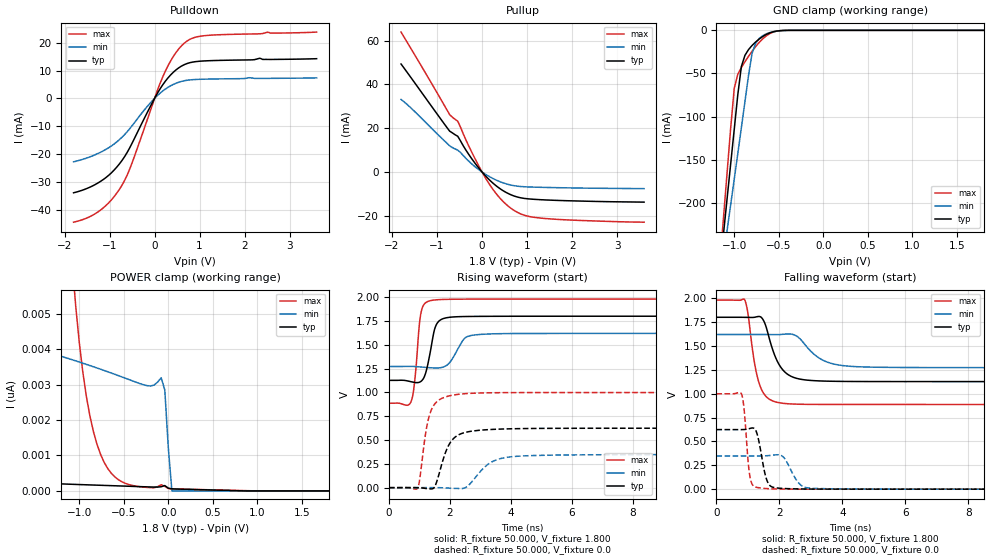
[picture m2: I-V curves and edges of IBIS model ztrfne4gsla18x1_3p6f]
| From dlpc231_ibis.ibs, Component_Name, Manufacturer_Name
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| Model ztrfne4gsla18x1_3p6f
[Model] ztrfne4gsla18x1_3p6f
Model_type I/O
Polarity   Non-Inverting
Enable   Active-High
Vinl =  0.540V
Vinh =  1.260V
Vref = 0.000V
Rref = 0.50k
Cref = 50.00pF
Vmeas = 0.90V
C_comp   2.222pF   2.219pF   2.262pF
C_comp_pullup   0.543pF   0.497pF   0.685pF
C_comp_pulldown   0.543pF   0.497pF   0.685pF
[Temperature Range]   25.000   0.125k   -40.000
[Voltage Range]   1.800V   1.620V   1.980V
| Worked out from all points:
|   slope of the pulldown table from 0 to 0.27 V, typ, clamps not added: 39.8 ohm
|   slope of the pullup table from 0 to 0.27 V, typ, clamps not added: 48.5 ohm
|   GND clamp passes 1 mA (typ) near -0.53 V on its own axis
|   rising waveform, R_fixture 50.000, V_fixture 1.800: 20-80 % time 249ps typ, 379ps min, 175ps max; typ from 1.13 V to 1.8 V
|   rising waveform, R_fixture 50.000, V_fixture 0.0: 20-80 % time 444ps typ, 682ps min, 315ps max; typ from 0 V to 0.624 V
|   falling waveform, R_fixture 50.000, V_fixture 1.800: 20-80 % time 472ps typ, 720ps min, 326ps max; typ from 1.8 V to 1.13 V
|   falling waveform, R_fixture 50.000, V_fixture 0.0: 20-80 % time 222ps typ, 355ps min, 145ps max; typ from 0.624 V to 0 V
[Pulldown]
-1.8V     -33.89mA   -22.78mA   -44.44mA
-1.2V     -29.79mA   -19.34mA   -40.09mA
-960mV    -26.74mA   -17.1mA    -36.45mA
-720mV    -22.21mA   -13.88mA   -31.07mA
-540mV    -17.37mA   -10.64mA   -24.87mA
-120mV    -3.725mA   -2.11mA    -5.686mA
180mV     4.844mA    2.631mA    7.654mA
420mV     9.436mA    5.045mA    15.14mA
660mV     12.11mA    6.338mA    19.82mA
840mV     13.02mA    6.716mA    21.6mA
1.14V     13.48mA    6.915mA    22.56mA
3.6V      14.25mA    7.361mA    23.8mA
[Pullup]
-1.8V     49.28mA    33.12mA    63.84mA
-1.56V    42.51mA    28.83mA    55.63mA
-720mV    18.65mA    11.97mA    26.18mA
-540mV    16.3mA     9.959mA    23.16mA
-300mV    8.153mA    5.032mA    12.05mA
-60mV     1.481mA    878.9uA    2.274mA
240mV     -5.044mA   -2.946mA   -7.881mA
420mV     -7.9mA     -4.584mA   -12.43mA
600mV     -10mA      -5.745mA   -15.9mA
900mV     -11.92mA   -6.675mA   -19.45mA
1.26V     -12.58mA   -6.952mA   -20.92mA
3.6V      -13.74mA   -7.586mA   -22.89mA
[GND_clamp]
-1.8V     -927mA     -775.7mA   -1.101A
-1.16V    -275.3mA   -291.3mA   -268.1mA
-1.12V    -235.1mA   -261.5mA   -216.5mA
-1.08V    -194.9mA   -231.7mA   -164.9mA
-1V       -114.9mA   -172.5mA   -67.23mA
-920mV    -41.99mA   -112.9mA   -43.08mA
-880mV    -29.06mA   -82.77mA   -36.47mA
-800mV    -17.56mA   -26.87mA   -24.31mA
-760mV    -13.55mA   -15.08mA   -18.89mA
-680mV    -7.158mA   -6.178mA   -9.822mA
-440mV    -133.7uA   -176.5uA   -112.6uA
1.8V      0A         0A         0A
[POWER_clamp]
-1.8V     288.6pA    4.231nA    140.6nA
-1.08V    187.2pA    3.703nA    6.484nA
-1.04V    183.6pA    3.671nA    5.234nA
-960mV    176.5pA    3.605nA    3.359nA
-840mV    166pA      3.504nA    1.668nA
-720mV    155.7pA    3.399nA    806.1pA
-560mV    142pA      3.253nA    315.8pA
-200mV    111.6pA    2.962nA    92.54pA
-80mV     117.3pA    3.191nA    175.1pA
-40mV     151.6pA    2.851nA    129.2pA
40mV      60.08pA    0A         58.67pA
1.8V      0A         0A         0A
[Ramp]
dV/dt_r   0.374/0.449n   0.209/0.692n   0.599/0.319n
dV/dt_f   0.404/0.469n   0.209/0.717n   0.656/0.329n
R_load = 50.000
[Rising Waveform]
R_fixture= 50.000
V_fixture= 1.800
V_fixture_min= 1.620
V_fixture_max= 1.980
0s        1.127V     1.272V     886.8mV
730ps     1.112V     1.273V     906.8mV
829ps     1.106V     1.272V     1.073V
1.05ns    1.116V     1.267V     1.833V
1.36ns    1.432V     1.259V     1.963V
1.58ns    1.725V     1.256V     1.973V
2.095ns   1.792V     1.361V     1.978V
2.485ns   1.797V     1.569V     1.979V
3.02ns    1.798V     1.609V     1.98V
15ns      1.8V       1.62V      1.98V
[Rising Waveform]
R_fixture= 50.000
V_fixture= 0.0
V_fixture_min= 0.0
V_fixture_max= 0.0
0s        0V         0V         0V
930ps     -179.7uV   489.9uV    -9.131mV
1.229ns   -9.268mV   501.5uV    618.9mV
1.35ns    -12.53mV   431.1uV    781.5mV
1.531ns   30.72mV    100.2uV    889.7mV
2.021ns   478.2mV    -5.753mV   966.7mV
2.51ns    580.6mV    -73.55uV   986.9mV
3.311ns   610.1mV    258.9mV    995.9mV
4.151ns   619mV      328.5mV    997.9mV
15ns      623.9mV    347.9mV    998.7mV
[Falling Waveform]
R_fixture= 50.000
V_fixture= 1.800
V_fixture_min= 1.620
V_fixture_max= 1.980
0s        1.8V       1.62V      1.98V
896ps     1.799V     1.62V      1.983V
996ps     1.799V     1.62V      1.854V
1.346ns   1.809V     1.62V      1.122V
1.534ns   1.741V     1.62V      987.7mV
1.926ns   1.346V     1.619V     910mV
2.518ns   1.164V     1.609V     890.5mV
3.277ns   1.134V     1.37V      887.4mV
4.248ns   1.128V     1.287V     887mV
15ns      1.127V     1.272V     886.8mV
[Falling Waveform]
R_fixture= 50.000
V_fixture= 0.0
V_fixture_min= 0.0
V_fixture_max= 0.0
0s        623.9mV    347.9mV    998.7mV
796ps     623.8mV    347.8mV    998.1mV
876ps     624.7mV    347.8mV    850mV
1.065ns   635.8mV    347.7mV    133.9mV
1.304ns   565.8mV    347.7mV    17.43mV
1.604ns   93.65mV    350.3mV    5.981mV
1.908ns   13.06mV    360.2mV    2.026mV
2.667ns   2.374mV    47.09mV    168.1uV
3.017ns   1.209mV    9.605mV    56.36uV
15ns      0V         0V         0V
